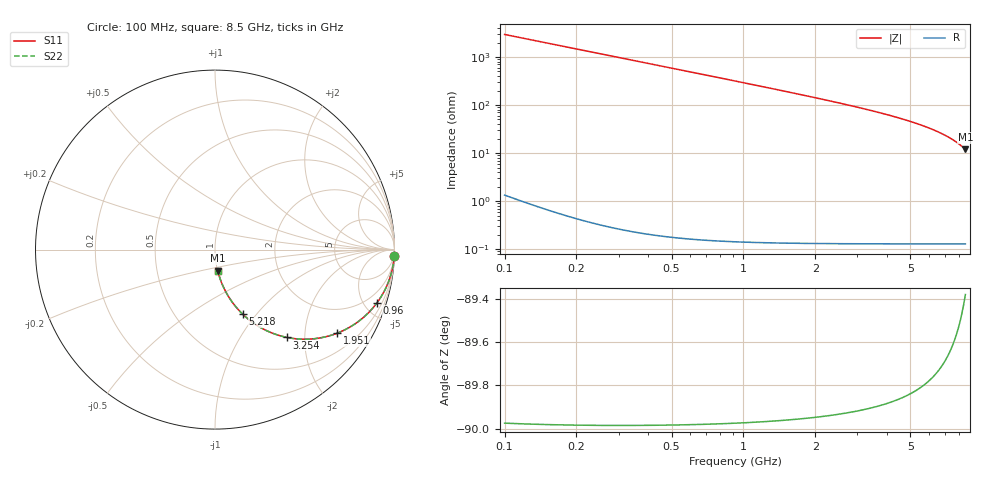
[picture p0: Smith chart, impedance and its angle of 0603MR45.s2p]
! Created Wed Apr 18 16:58:25 2012
# hz S ma R 50
! 2 Port Network Data from SP1.SP block
! freq  magS11  angS11  magS21  angS21  magS12  angS12  magS22  angS22
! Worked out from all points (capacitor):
!   8401 points, 100 MHz to 8.5 GHz, reference 50 ohm
!   read as one part in series: C = 540 fF near 142 MHz
!   lowest |Z| = 11.9 ohm at 8.5 GHz (marker M1)
!   S11 on the Smith chart (normalised r, x): 100 MHz: 1, -59; 960 MHz: 1.00, -6.09; 1.951 GHz: 1.00, -2.92; 3.254 GHz: 1.00, -1.64; 5.218 GHz: 1.00, -0.85; 8.5 GHz: 1.00, -0.24
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1e8  0.9994 -1.9  0.03391 88.0  0.03391 88.0  0.9994 -1.9
1.25e8  0.9991 -2.4  0.04238 87.5  0.04238 87.5  0.9991 -2.4
1.82e8  0.9981 -3.5  0.06165 86.4  0.06165 86.4  0.9981 -3.5
2.35e8  0.9968 -4.6  0.07952 85.4  0.07952 85.4  0.9968 -4.6
3.1e8  0.9945 -6.0  0.1047 84.0  0.1047 84.0  0.9945 -6.0
4e8  0.9909 -7.7  0.1347 82.2  0.1347 82.2  0.9909 -7.7
5.11e8  0.9852 -9.9  0.1712 80.1  0.1712 80.1  0.9852 -9.9
6.41e8  0.9769 -12.3  0.2133 77.7  0.2133 77.7  0.9769 -12.3
7.9e8  0.9654 -15.1  0.2602 74.9  0.2602 74.9  0.9654 -15.1
9.6e8  0.9499 -18.2  0.312 71.8  0.312 71.8  0.9499 -18.2
1.211e9  0.923 -22.6  0.3843 67.4  0.3843 67.4  0.923 -22.6
1.5e9  0.8871 -27.4  0.4609 62.5  0.4609 62.5  0.8871 -27.4
1.951e9  0.8244 -34.4  0.5652 55.5  0.5652 55.5  0.8244 -34.4
2.401e9  0.7579 -40.7  0.6515 49.3  0.6515 49.3  0.7579 -40.7
2.9e9  0.684 -46.8  0.7285 43.2  0.7285 43.2  0.684 -46.8
3.254e9  0.6331 -50.6  0.7731 39.3  0.7731 39.3  0.6331 -50.6
4.3e9  0.4951 -60.2  0.8677 29.7  0.8677 29.7  0.4951 -60.2
5.218e9  0.391 -66.8  0.9192 23.0  0.9192 23.0  0.391 -66.8
5.7e9  0.3422 -69.8  0.9384 20.0  0.9384 20.0  0.3422 -69.8
7.1e9  0.2192 -77.0  0.9744 12.7  0.9744 12.7  0.2192 -77.0
7.835e9  0.1637 -80.1  0.9852 9.4  0.9852 9.4  0.1637 -80.1
8.5e9  0.1177 -82.6  0.9918 6.8  0.9918 6.8  0.1177 -82.6
